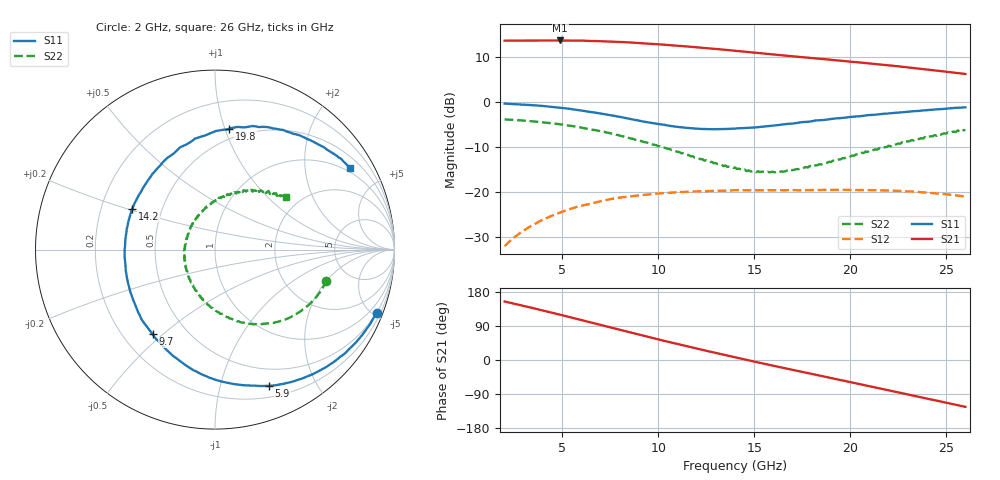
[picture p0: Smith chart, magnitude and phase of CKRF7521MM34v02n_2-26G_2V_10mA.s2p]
! CHUO DENSHI KOGYO Co.,Ltd.
! 2. June 2016
! CKRF7521MM34
! N-channel HJ-FET
! Vds = 2 V Id = 10 mA
# Hz S  MA  R 50
!  f  S11  S21  S12  S22
!  Hz  MAG  ANG  MAG  ANG  MAG  ANG  MAG  ANG
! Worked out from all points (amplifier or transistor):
!   241 points, 2 GHz to 26 GHz, reference 50 ohm
!   highest |S21| = 13.7 dB at 4.9 GHz (marker M1)
!   |S21| within 3 dB of that: start of sweep to 15.73 GHz
!   unconditionally stable (mu >= 1): 13.42 GHz to 19.2 GHz
!   at 6 GHz: K = 0.54, MSG = 18.3 dB, |S12| = -23.0 dB
!   at 14 GHz: K = 1.01, MAG = 15.0 dB, |S12| = -19.5 dB
!   at 26 GHz: K = 0.68, MSG = 13.6 dB, |S12| = -20.9 dB
!   lowest NFmin = 0.69 dB at 18 GHz
!   S11 on the Smith chart (normalised r, x): 2 GHz: 0.50, -5.28; 5.9 GHz: 0.31, -1.43; 9.7 GHz: 0.32, -0.46; 14.2 GHz: 0.34, +0.21; 19.8 GHz: 0.42, +1.03; 26 GHz: 0.86, +3.40
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2e9  0.9663 -21.3  4.828 154.4  0.02526 73.8  0.6447 -15.5
3.5e9  0.9277 -38.1  4.844 136.6  0.0437 62.8  0.6125 -28.3
4.9e9  0.87 -55.1  4.855 119.4  0.05986 52.4  0.5684 -40.7
5.9e9  0.8169 -68.3  4.841 106.5  0.07009 44.3  0.5271 -50.0
6e9  0.8101 -69.7  4.833 105.2  0.07099 43.5  0.5242 -51.2
7e9  0.7505 -83.4  4.765 92.4  0.07969 36.4  0.4782 -60.7
7.8e9  0.7013 -95.5  4.704 82.1  0.0859 30.3  0.4355 -68.8
8.8e9  0.6375 -111.3  4.578 69.3  0.09149 23.2  0.3837 -78.8
9.7e9  0.5862 -126.3  4.446 58.1  0.09579 17.4  0.3408 -89.3
1e10  0.5736 -131.3  4.406 54.4  0.09715 15.5  0.3255 -92.5
1.09e10  0.5358 -147.7  4.257 43.4  0.09981 9.9  0.2867 -104.1
1.19e10  0.5113 -166.1  4.095 31.4  0.1023 4.2  0.2432 -117.9
1.29e10  0.502 176.0  3.928 19.7  0.104 -1.0  0.2102 -133.4
1.4e10  0.5099 156.9  3.731 7.0  0.1057 -6.4  0.1885 -153.7
1.42e10  0.5137 153.7  3.696 4.8  0.106 -7.5  0.183 -157.0
1.6e10  0.5513 127.0  3.395 -15.3  0.1056 -15.6  0.1685 164.3
1.8e10  0.6159 102.5  3.098 -36.6  0.106 -23.7  0.1921 126.8
1.98e10  0.6768 83.3  2.853 -56.2  0.1065 -31.7  0.2457 100.6
2.09e10  0.7186 73.3  2.711 -68.1  0.1058 -36.7  0.2802 86.2
2.2e10  0.7525 63.6  2.564 -80.0  0.1045 -42.3  0.3289 72.8
2.37e10  0.8077 49.1  2.348 -98.6  0.1003 -51.1  0.3996 54.9
2.6e10  0.8783 31.1  2.06 -123.6  0.08969 -63.2  0.4915 36.6
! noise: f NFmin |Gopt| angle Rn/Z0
1.8e+10  0.695  0.447  -117  0.09
1.85e+10  0.705  0.462  -109.9  0.1
1.9e+10  0.715  0.478  -103.1  0.116
2e+10  0.73  0.504  -89.67  0.156
2.05e+10  0.74  0.514  -85.72  0.179
2.1e+10  0.75  0.534  -79.94  0.205
2.2e+10  0.79  0.556  -70.11  0.261
2.25e+10  0.8  0.562  -65.87  0.295
2.3e+10  0.82  0.564  -59.84  0.332
2.4e+10  0.882  0.574  -50.62  0.404
